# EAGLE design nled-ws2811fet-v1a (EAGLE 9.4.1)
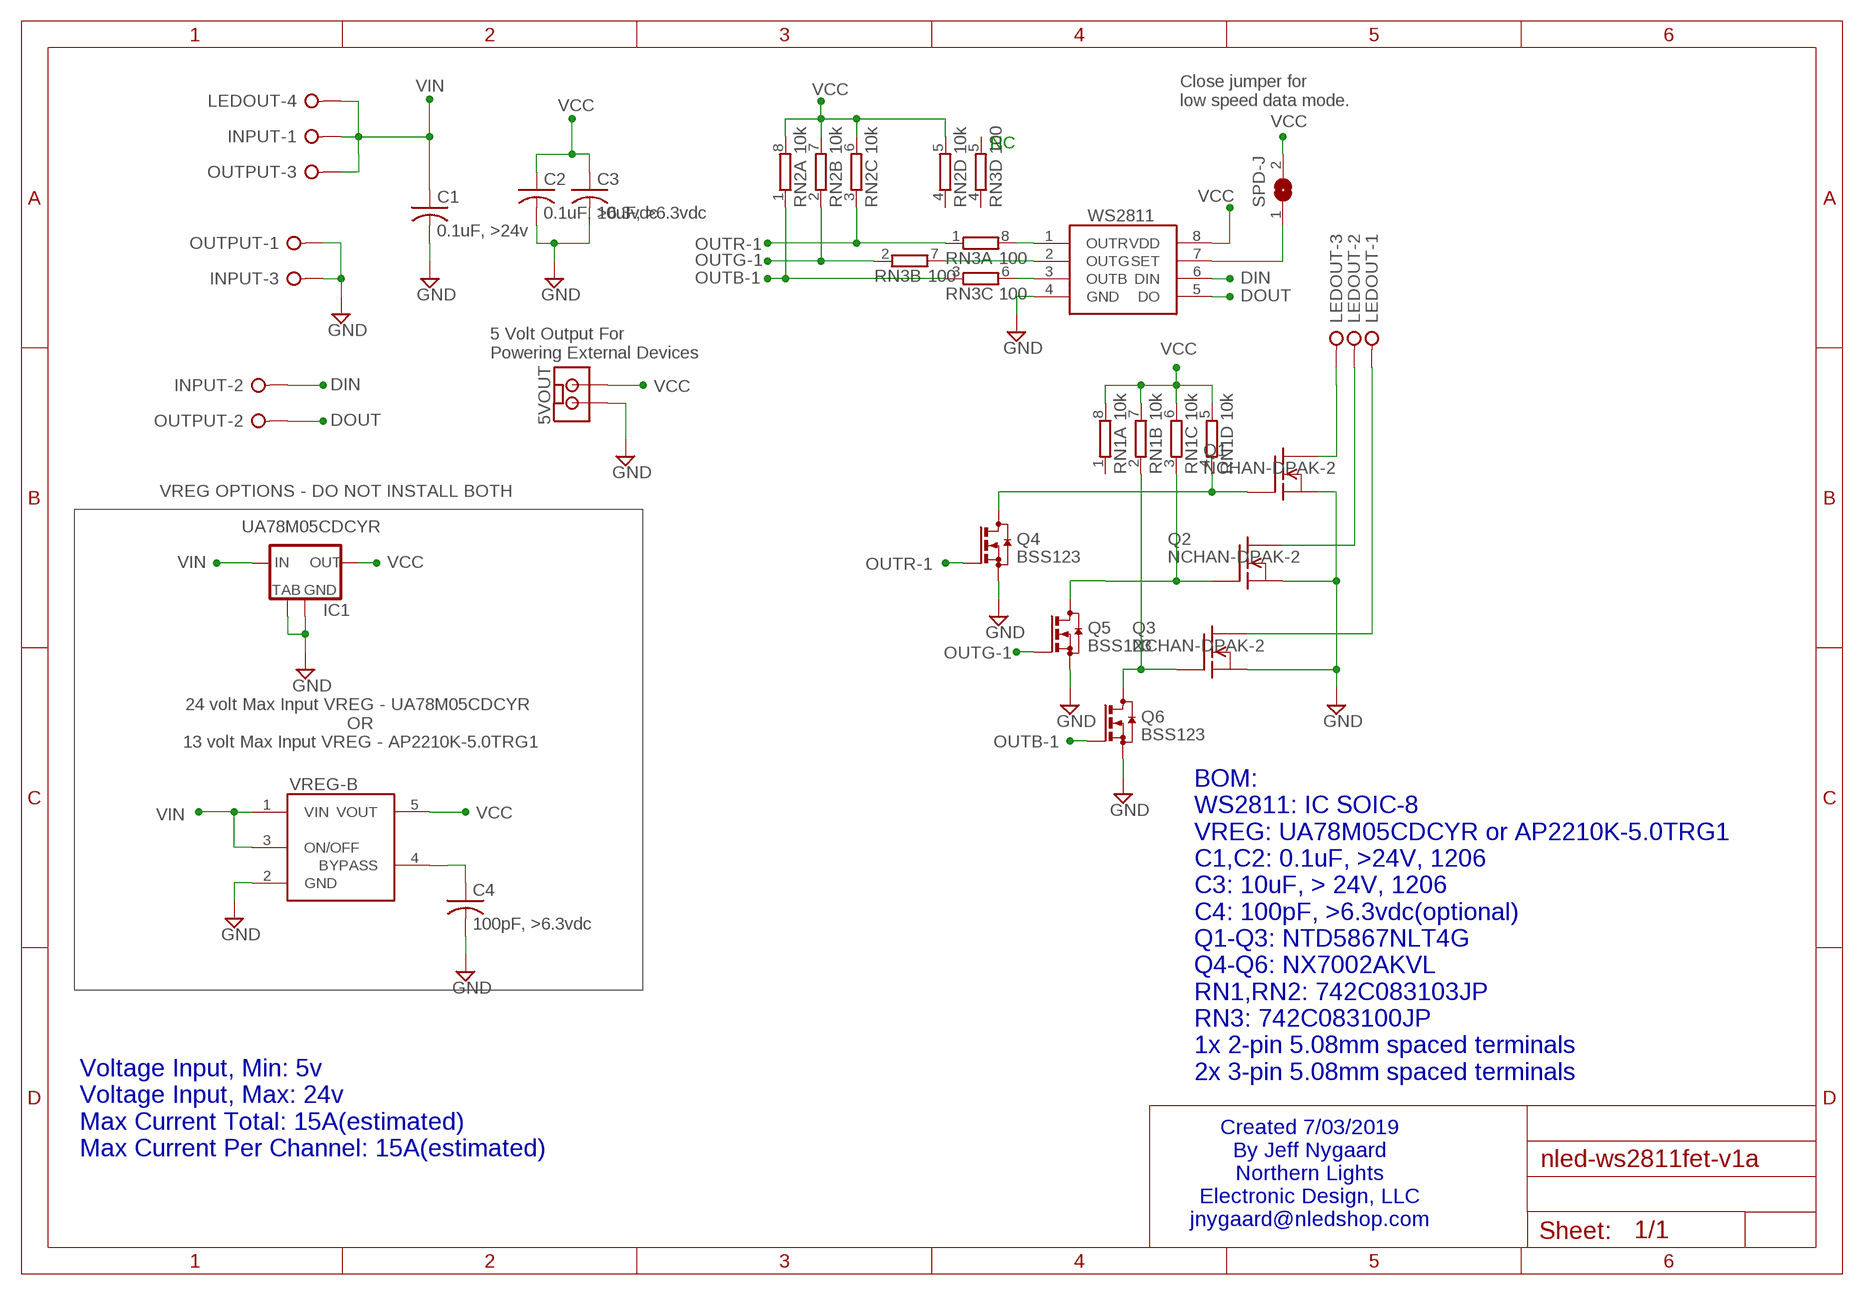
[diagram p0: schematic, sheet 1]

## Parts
5VOUT  MOLEX-KK-2PSM  [MOLEXKK2PWR-SM]
C1  0.1uF, >24v  C-USC1206  [C1206]
C2  0.1uF, >6.3vdc  C-USC1206  [C1206]
C3  10uF, >6.3vdc  C-USC1206  [C1206]
C4  100pF, >6.3vdc  C-USC0805  [C0805]
IC1  MCP1703/UA78M00  [SOT223]
INPUT  W237-03P  [W237-133]
LEDOUT  W237-04P  [W237-4P]
OUTPUT  W237-03P  [W237-133]
Q1  NCHAN-DPAK-2  [DPAK-2PIN]
Q2  NCHAN-DPAK-2  [DPAK-2PIN]
Q3  NCHAN-DPAK-2  [DPAK-2PIN]
Q4  BSS123  [SOT23]
Q5  BSS123  [SOT23]
Q6  BSS123  [SOT23]
RN1  10k  4R-N0603-ARV  [0603-ARV]
RN2  10k  4R-N0603-ARV  [0603-ARV]
RN3  100  4R-N0603-ARV  [0603-ARV]
SPD-J  SJ  [SJ]
VREG-B  AP2210K  [SOT25]
WS2811  WS2811  [SOIC-8]

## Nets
BINV: Q3.1(G) Q6.3(D) RN1.2
BYPASS: C4.1 VREG-B.4(BYPASS)
DIN: INPUT.2 WS2811.6(DIN)
DOUT: OUTPUT.2 WS2811.5(DO)
GINV: Q2.1(G) Q5.3(D) RN1.3
GND: 5VOUT.2 C1.2 C2.2 C3.2 C4.2 IC1.2(GND) IC1.4(TAB) INPUT.3 OUTPUT.1 Q1.3(S) Q2.3(S) Q3.3(S) Q4.2(S) Q5.2(S) Q6.2(S) VREG-B.2(GND) WS2811.4(GND)
N$3: RN3.8 WS2811.1(OUTR)
N$5: RN3.7 WS2811.2(OUTG)
N$7: RN3.6 WS2811.3(OUTB)
N$13: SPD-J.1 WS2811.7(SET)
OUTB-1: Q6.1(G) RN2.1 RN3.3
OUTBLUE: LEDOUT.3 Q1.2(D)
OUTG-1: Q5.1(G) RN2.2 RN3.2
OUTGREEN: LEDOUT.2 Q2.2(D)
OUTR-1: Q4.1(G) RN2.3 RN3.1
OUTRED: LEDOUT.1 Q3.2(D)
RINV: Q1.1(G) Q4.3(D) RN1.4
VCC: 5VOUT.1 C2.1 C3.1 IC1.3(OUT) RN1.5 RN1.6 RN1.7 RN1.8 RN2.5 RN2.6 RN2.7 RN2.8 SPD-J.2 VREG-B.5(VOUT) WS2811.8(VDD)
VIN: C1.1 IC1.1(IN) INPUT.1 LEDOUT.4 OUTPUT.3 VREG-B.1(VIN) VREG-B.3(ON/OFF)
Unconnected: RN1.1 RN2.4 RN3.4 RN3.5

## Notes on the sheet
- Close jumper for
  low speed data mode.
- NC
- 5 Volt Output For
  Powering External Devices
- VREG OPTIONS - DO NOT INSTALL BOTH
- UA78M05CDCYR
- 24 volt Max Input VREG - UA78M05CDCYR 
  OR
  13 volt Max Input VREG - AP2210K-5.0TRG1
- BOM:
  WS2811: IC SOIC-8
  VREG: UA78M05CDCYR or AP2210K-5.0TRG1
  C1,C2: 0.1uF, >24V, 1206
  C3: 10uF, > 24V, 1206
  C4: 100pF, >6.3vdc(optional)
  Q1-Q3: NTD5867NLT4G
  Q4-Q6: NX7002AKVL
  RN1,RN2: 742C083103JP 
  RN3: 742C083100JP
  1x 2-pin 5.08mm spaced terminals
  2x 3-pin 5.08mm spaced terminals
- Voltage Input, Min: 5v
  Voltage Input, Max: 24v
  Max Current Total: 15A(estimated)
  Max Current Per Channel: 15A(estimated)
- Created 7/03/2019
  By Jeff Nygaard
  Northern Lights
  Electronic Design, LLC
  jnygaard@nledshop.com

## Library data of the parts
5VOUT = NLED-connectors:MOLEX-KK-2P
C1-C3 = rcl:C-US: CAPACITOR, American symbol
C4 = rcl:C-US: CAPACITOR, American symbol; SPICEPREFIX: C
IC1 = NLED-integratedcircuit:MCP1703/UA78M00: VOLTAGE REGULATOR
INPUT OUTPUT = con-wago-508:W237-03P: WAGO SREW CLAMP; OC_FARNELL: unknown; OC_NEWARK: unknown
LEDOUT = con-wago-508:W237-04P: WAGO SREW CLAMP; OC_FARNELL: unknown; OC_NEWARK: unknown
Q1-Q3 = NLED-integratedcircuit:NCHAN-DPAK-2
Q4-Q6 = transistor-small-signal:BSS123: N-CHANNEL MOS FET
RN1-RN3 = resistor-dil:4R-N: Array Chip Resistor Source: RS Component / Phycomp; OC_FARNELL: unknown; OC_NEWARK: unknown
SPD-J = NLED-misc:SJ: SMD solder JUMPER
VREG-B = NLED-integratedcircuit:AP2210K: AP2210K - Diodes Incorporated LDO Voltage Regulators 300mA CMOS LDO 5.0V 250mV
WS2811 = NLED-integratedcircuit:WS2811

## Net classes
0 default: width 0.406 mm

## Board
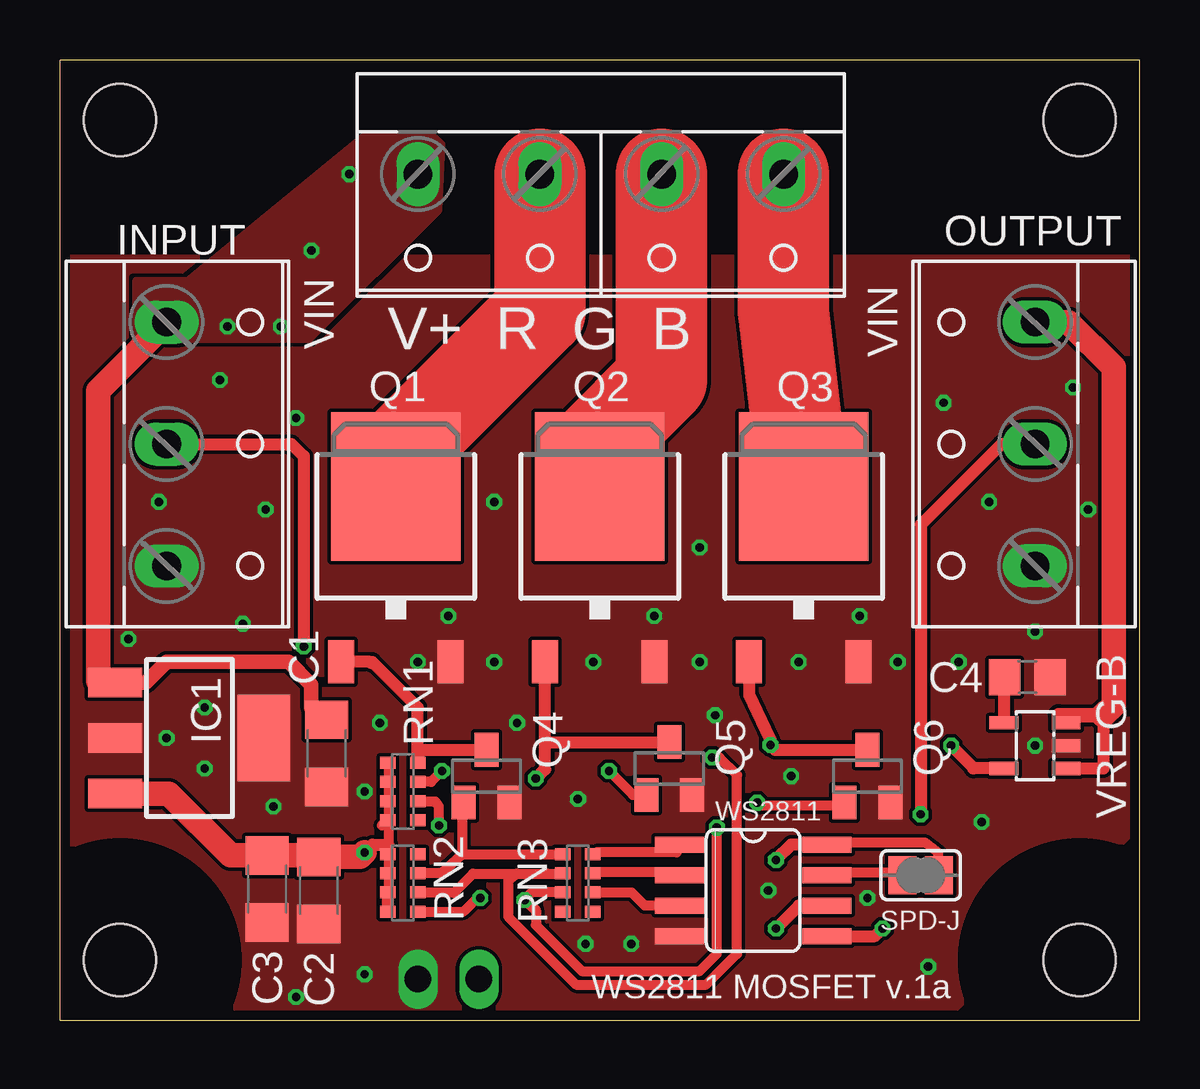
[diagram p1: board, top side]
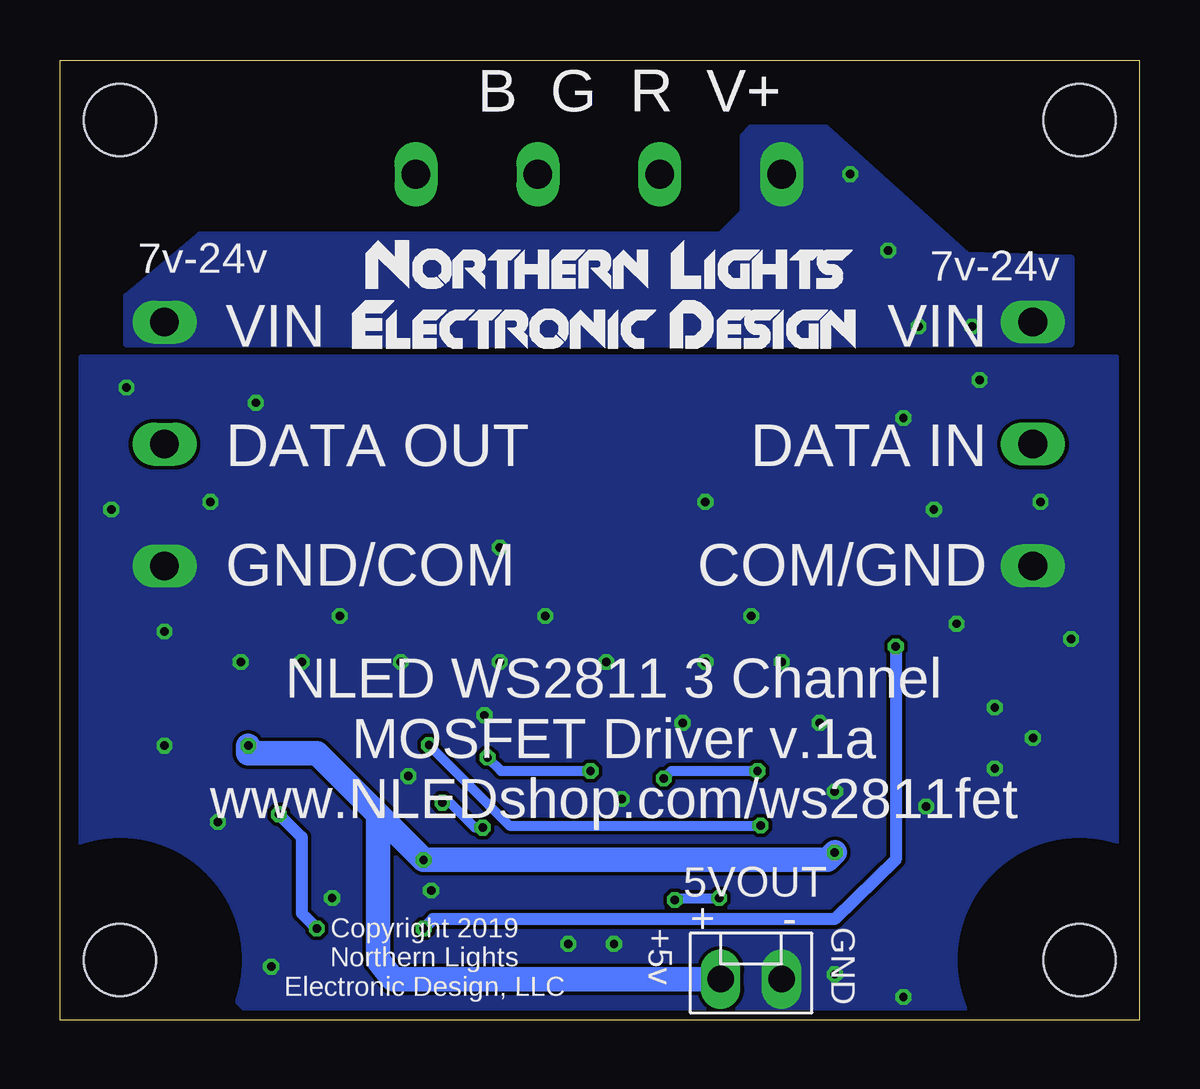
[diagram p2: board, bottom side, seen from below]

Size 45 x 40 mm. Coordinates in mm from the lower left corner, seen from the top.
Outline: 0,0 45,0 45,40 0,40 0,0
Copper layers (1*2*15*16): Top 0.035mm / dielectric 0.2mm / Route2 0.0175mm / dielectric 1.1mm / Route15 0.0175mm / dielectric 0.2mm / Bottom 0.035mm
Design rules "SeeedStudio_DRU_no_angle_20130527 *": minimum track width 6mil, minimum drill 12mil, track to track 6mil, track to pad 12mil, pad to pad 6mil, via to via 6mil, smd to smd 0mil, copper to edge 16mil, drill to drill 10mil, minimum pad ring 6mil, minimum via ring 6mil, stop-mask expansion 2mil, vias tented up to drill 25mil, thermal gap 10mil
Holes 3 mm at 2.5,2.5 42.5,37.5 2.5,37.5 42.5,2.5
tRestrict: area -2.5,32.5 to 7.5,42.5; area -2.5,-2.5 to 7.5,7.5; area 37.5,32.5 to 47.5,42.5; area 37.5,-2.5 to 47.5,7.5
bRestrict: area -2.5,-2.5 to 7.5,7.5; area -2.5,32.5 to 7.5,42.5; area 37.5,32.5 to 47.5,42.5; area 37.5,-2.5 to 47.5,7.5

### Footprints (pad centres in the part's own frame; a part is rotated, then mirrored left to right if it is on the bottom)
MOLEXKK2PWR-SM = drill 1.1 long: 1 -1.27,0; 2 1.27,0
C1206 = smd 1.6 x 1.8: 1 -1.4,0; 2 1.4,0
C0805 = smd 1.3 x 1.5: 1 -0.95,0; 2 0.95,0
SOT223 = smd 1.219 x 2.235: 1 -2.311,-3.099; 2 0,-3.099; 3 2.311,-3.099 | smd 3.6 x 2.2: 4 0,3.099
W237-133 = drill 1.194 long: 1 -5.08,-0.635; 2 0,-0.635; 3 5.08,-0.635
W237-4P = drill 1.194 long: 1 -7.62,-0.635; 2 -2.54,-0.635; 3 2.54,-0.635; 4 7.62,-0.635
DPAK-2PIN = smd 1.067 x 1.778: 1 -2.28,-6.07; 3 2.28,-6.07 | smd 5.4 x 6.2: 2 0,1.23
SOT23 = smd 1 x 1.4: 1 -0.95,-1.1; 2 0.95,-1.1; 3 0,1.1
0603-ARV = smd 0.5 x 0.65: 1 -1.2,-0.625; 2 -0.4,-0.625; 3 0.4,-0.625; 4 1.2,-0.625; 5 1.2,0.625; 6 0.4,0.625; 7 -0.4,0.625; 8 -1.2,0.625
SJ = smd 1.168 x 1.6: 1 -0.762,0; 2 0.762,0
SOT25 = smd 0.55 x 1.2: 1 -0.95,-1.3; 2 0,-1.3; 3 0.95,-1.3; 4 0.95,1.3; 5 -0.95,1.3
SOIC-8 = smd 0.66 x 2.032: 1 -1.905,-3.073; 2 -0.635,-3.073; 3 0.635,-3.073; 4 1.905,-3.073; 5 1.905,3.073; 6 0.635,3.073; 7 -0.635,3.073; 8 -1.905,3.073

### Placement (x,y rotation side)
5VOUT  16.19,1.7 0 bottom
C1  11.11,11.11 270 top
C2  10.79,5.4 270 top
C3  8.64,5.46 270 top
C4  40.32,14.29 0 top
IC1  5.4,11.75 270 top
INPUT  5.08,24 270 top
LEDOUT  22.54,34.61 180 top
OUTPUT  40.01,24 90 top
Q1  14,21 0 top
Q2  22.5,21 0 top
Q3  31,21 0 top
Q4  17.78,10.16 0 top
Q5  25.4,10.48 0 top
Q6  33.66,10.16 0 top
RN1  14.29,9.53 90 top
RN2  14.29,5.71 90 top
RN3  21.59,5.71 270 top
SPD-J  35.88,6.03 0 top
VREG-B  40.64,11.43 90 top
WS2811  28.89,5.4 270 top

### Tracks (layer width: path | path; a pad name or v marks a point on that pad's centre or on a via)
BINV  (via drill 0.35)
  Top 0.406: RN1.2 15.05,9.1 15.65,9.1 15.8,8.9 v15.8,8.1
  Top 0.508: Q3.1 28.72,13.59 29.62,11.69 v29.62,11.46 29.81,11.26 Q6.3
  Bottom 0.406: v15.8,8.1 26.26,8.1 v29.62,11.46
BYPASS
  Top 0.508: VREG-B.4 39.37,12.41 C4.1
DIN  (via drill 0.35)
  Top 0.508: WS2811.6 30.8,4.76 v29.84,3.81 | v10.16,15.56 10.16,23.5 9.65,24 INPUT.2
  Bottom 0.508: v10.16,15.56 10.16,6.67 12.7,4.2 25.08,4.2 29.45,4.2 v29.84,3.81
DOUT  (via drill 0.35)
  Top 0.508: WS2811.5 33.97,3.49 v34.29,3.81 | OUTPUT.2 39.24,24 35.88,20.64 v35.88,8.57
  Bottom 0.508: v34.29,3.81 34.92,4.45 34.92,7.62 v35.88,8.57
GINV  (via drill 0.35)
  Top 0.406: v15.93,10.38 15.47,9.93 RN1.3
  Top 0.508: v19.84,10.06 20.22,10.44 20.22,11.43 | 20.22,11.43 Q2.1 | 20.22,11.43 20.37,11.58 Q5.3
  Bottom 0.406: v19.84,10.06 19.52,10.38 v15.93,10.38
GND  (via drill 0.35)
  other vias: 18.1,21.59 4.13,21.59 19.05,12.38 9.84,0.95 2.86,15.88 4.45,11.75 36.83,25.72 9.84,25.08 38.42,8.26 37.47,14.92 12.7,1.91 21.91,3.17 23.81,3.17 21.59,9.21 27.3,12.7 30.48,10.16 38.73,21.59 40.64,11.43 26.67,19.68 40.64,16.19 13.34,12.38 8.89,8.89 6.03,10.48 7.62,16.51 8.57,21.27 22.23,14.92 26.67,14.92 14.92,14.92 30.8,14.92 34.92,14.92 33.34,16.83 24.77,16.83 16.19,16.83 18.1,14.92 33.66,5.08 29.53,5.4 12.7,9.53 6.03,13.02 6.67,26.67 42.23,26.35 42.86,21.27 36.2,2.22
  pour Top (rank 2, no thermals): 0,31.75 45.09,31.75 45.09,8.26 36.83,0 7.62,0 0,7.62
  pour Bottom (rank 2, no thermals): 0.95,27.62 44.13,27.62 44.13,7.3 36.83,0 7.62,0 0.95,6.67
N$3
  Top 0.406: RN3.8 22.35,6.99 25.7,6.99 WS2811.1
N$5
  Top 0.406: RN3.7 22.35,6.15 25.7,6.15 WS2811.2
N$7
  Top 0.406: WS2811.3 24.38,4.76 23.84,5.31 22.35,5.31 RN3.6
N$13
  Top 0.406: SPD-J.1 35.01,6.15 32.13,6.15 WS2811.7
OUTB-1  (via drill 0.35)
  Top 0.406: 32.69,8.94 Q6.1 32.69,8.94 | v17.53,5.08 17.52,5.22 16.82,4.51 RN2.1 | RN3.3 19.68,5.32 v19.37,5 19.84,4.58 19.84,3.95 21.75,2.03 26.66,2.03 27.38,2.76 v27.38,8.01 | 32.69,8.94 29.06,8.94 v29.06,9.05
  Bottom 0.406: v19.37,5 19.37,4.9 19.35,5.08 v17.53,5.08 | v29.06,9.05 28.74,9.05 27.7,8.01 v27.38,8.01
OUTBLUE
  Top 2.54: Q1.2 14.29,22.38 13.34,22.86
  Top 3.81: 13.34,22.86 20,29.53 LEDOUT.3
OUTG-1  (via drill 0.35)
  Top 0.406: RN2.2 14.98,5.3 16.42,5.3 17.21,6.1 19.05,6.1 | v22.89,10.38 23.88,9.38 Q5.1 | v27.18,10.94 27.5,10.94 28.22,10.21 28.22,2.76 26.94,1.47 21.51,1.47 18.68,4.3 18.68,5.81 19.05,6.1 | 19.05,6.1 20.32,6.1 | 20.32,6.1 20.72,6.1 | 20.32,6.1 RN3.2
  Bottom 0.406: v22.89,10.38 26.62,10.38 v27.18,10.94
OUTGREEN
  Top 3.81: LEDOUT.2 25.08,26.67 22.22,23.81 22.21,21.52 Q2.2
OUTR-1
  Top 0.406: 16.76,6.9 15.89,6.12 RN2.3 | 16.76,6.9 16.76,8.94 Q4.1 | 16.76,6.9 20.68,6.9 RN3.1
OUTRED
  Top 3.81: LEDOUT.1 30.16,29.53 Q3.2
RINV
  Top 0.508: Q1.1 12.87,14.93 12.98,14.88 13.02,14.92 14.91,13.03 RN1.4 14.91,11.04 15.13,11.26 Q4.3
VCC  (via drill 0.35)
  Top 0.406: 13.69,4.47 13.66,4.5 RN2.8 | RN2.7 13.68,5.32 13.69,5.31 13.69,5.94 RN2.6 13.69,6.14 13.69,6.15 13.69,6.78 RN2.5 13.69,7.06 13.69,7.3 13.69,8.1 RN1.8 | RN1.8 13.69,8.38 13.69,8.94 RN1.7 13.69,9.22 13.69,9.78 RN1.6 13.69,10.06 13.69,10.62 RN1.5 | 13.41,8.1 RN1.8 | SPD-J.2 36.6,6.11 36.6,6.99 36.04,7.4 32.13,7.4 WS2811.8
  Top 0.508: v12.7,6.99 13.02,7.3 13.69,7.3 | WS2811.8 30.48,7.3 v29.84,6.67 | VREG-B.5 38.08,10.48 38.07,10.48 38.07,10.51 v37.15,11.43 | RN2.7 RN2.8
  Top 1.016: 10.73,6.86 C2.1 12.51,6.8 v12.7,6.99 | 10.73,6.86 C3.1 | 10.73,6.86 7.11,6.86 4.53,9.44 IC1.3
  Bottom 1.016: v12.7,6.99 13.02,6.67 v29.84,6.67 31.91,8.73 | 31.91,8.73 34.29,11.11 37.15,11.11 v37.15,11.43 | 5VOUT.1 31.11,1.7 31.75,2.49 31.75,8.57 31.91,8.73
VIN  (via drill 0.35)
  Top 0.508: VREG-B.1 43.5,10.48 43.5,12.7 | VREG-B.3 41.62,12.7 | IC1.1 1.66,14.06 1.59,14.13 | 3.58,14.06
  Top 0.61: 41.62,12.7 43.5,12.7 | 3.58,14.06 4.45,14.92 9.53,14.92 10.48,13.97 10.48,13.02 10.98,12.51 C1.1 | 3.58,14.06 IC1.1
  Top 1.016: OUTPUT.3 42.04,29.08 43.92,27.2 43.92,13.12 43.5,12.7 | INPUT.1 1.59,26.22 1.59,14.13
  other vias: 12.06,35.24 9.21,28.89 10.48,32.07 6.99,28.89
  pour Top (no thermals): 3.17,30.8 5.31,30.8 12.7,36.87 15.55,36.83 15.9,36.48 15.77,33.73 10.39,28.36 3.17,28.36
  pour Bottom (no thermals): 2.86,28.18 2.86,31.75 7.2,31.87 13.06,37.15 16.19,37.15 16.51,36.83 16.51,33.66 17.46,32.7 39.18,32.7 42.23,30.16 42.23,28.18

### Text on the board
tNames: VIN | V+ R G B | VIN | WS2811 MOSFET v.1a
bNames: B G R V+ | 7v-24v | 7v-24v | VIN / DATA IN / COM/GND | VIN / DATA OUT / GND/COM | NLED WS2811 3 Channel / MOSFET Driver v.1a / www.NLEDshop.com/ws2811fet | +5v | Copyright 2019 / Northern Lights / Electronic Design, LLC | GND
